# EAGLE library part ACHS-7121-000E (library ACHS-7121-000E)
Board Mount Current Sensors Hall Effect IC LF 10A 185mV/A Source: Datasheet
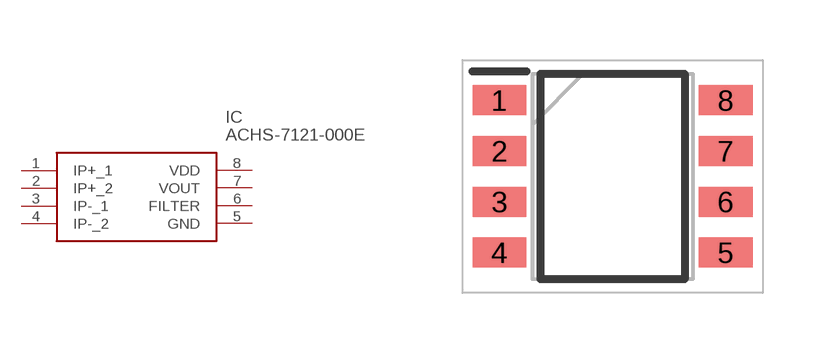
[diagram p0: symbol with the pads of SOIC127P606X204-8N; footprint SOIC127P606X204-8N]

Designator prefix IC

## ACHS-7121-000E (Description: Board Mount Current Sensors Hall Effect IC LF 10A 185mV/A; Height: 2.035mm; Manufacturer_Name: Avago Technologies; Manufacturer_Part_Number: ACHS-7121-000E; Mouser_Part_Number: 630-ACHS-7121-000E; Mouser_Price-Stock: https://www.mouser.co.uk/ProductDetail/Broadcom-Avago/ACHS-7121-000E?qs=w%2Fv1CP2dgqo3exDSmSklAg%3D%3D)  [SOIC127P606X204-8N]
1  IP+_1
2  IP+_2
3  IP-_1
4  IP-_2
5  GND
6  FILTER
7  VOUT
8  VDD

## Footprint SOIC127P606X204-8N (pad centres in mm)
ACHS-7121-000E
smd 1.35 x 0.75: 1 -2.825,1.905; 2 -2.825,0.635; 3 -2.825,-0.635; 4 -2.825,-1.905; 5 2.825,-1.905; 6 2.825,-0.635; 7 2.825,0.635; 8 2.825,1.905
